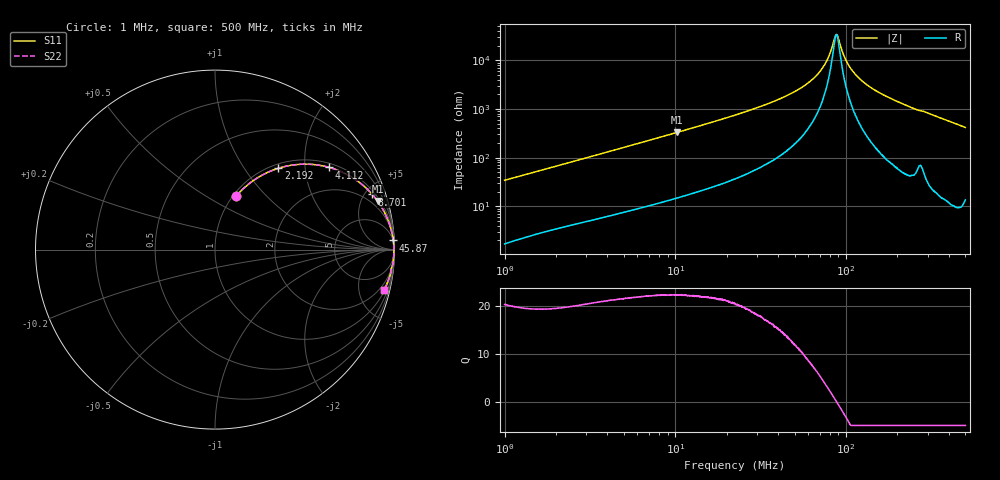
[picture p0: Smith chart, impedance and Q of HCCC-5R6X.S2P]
!s-Parameter Generated by FASTRON Sdn. Bhd.
!FASTRON P/N : HCCC-5R6X
!Keysight Technologies,E4991B,MY54100416,A.01.15
!Date: Thu Apr 02 15:32:48 2026
!Version  : Rev00 Thu Apr 02 15:32:48 2026
!Data & Calibration Information:
!PortZ  Port1:50+j0  Port2:50+j0
!When reading, reference impedance value at option line is always used.
! Remarks : This data is being provided solely for informational purposes.
!Freq	S11	S21	S12	S22
# Hz S dB R 50
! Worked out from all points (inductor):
!   1601 points, 1 MHz to 500 MHz, reference 50 ohm
!   read as one part in series: L = 5.38 uH near 1.032 MHz
!   highest Q = 22.3 at 10.24 MHz (marker M1), where L = 5.12 uH
!   self-resonance near 87.75 MHz
!   S11 on the Smith chart (normalised r, x): 1 MHz: 1.03, +0.68; 2.192 MHz: 1.07, +1.45; 4.112 MHz: 1.13, +2.68; 8.701 MHz: 1.25, +5.60; 45.87 MHz: 4, +39; 500 MHz: 1.27, -8.34
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1000000  -9.92 68.6  -0.61 -18.6  -0.61 -18.6  -9.92 68.6
2191518  -4.81 52.1  -2.05 -35.0  -2.05 -35.0  -4.81 52.1
2820919  -3.55 45.6  -2.91 -41.6  -2.91 -41.6  -3.55 45.6
4111646  -2.11 35.8  -4.66 -51.5  -4.66 -51.5  -2.11 35.8
7957584  -0.74 21.0  -8.92 -66.5  -8.92 -66.5  -0.74 21.0
8701196  -0.64 19.3  -9.59 -68.1  -9.59 -68.1  -0.64 19.3
1.024299e7  -0.49 16.6  -10.85 -70.8  -10.85 -70.8  -0.49 16.6
2.236068e7  -0.13 7.6  -17.60 -79.6  -17.60 -79.6  -0.13 7.6
4.587261e7  -0.05 2.9  -25.82 -82.7  -25.82 -82.7  -0.05 2.9
6.307767e7  -0.03 1.4  -31.99 -81.2  -31.99 -81.2  -0.03 1.4
6.978047e7  -0.03 1.0  -35.15 -78.6  -35.15 -78.6  -0.03 1.0
7.541731e7  -0.03 0.7  -38.55 -74.2  -38.55 -74.2  -0.03 0.7
7.994179e7  -0.03 0.4  -42.29 -66.3  -42.29 -66.3  -0.03 0.4
8.573088e7  -0.03 0.1  -49.11 -32.1  -49.11 -32.1  -0.03 0.1
8.809378e7  -0.03 -0.0  -50.64 3.7  -50.64 3.7  -0.03 -0.0
9.01709e7  -0.03 -0.1  -48.92 33.1  -48.92 33.1  -0.03 -0.1
1.001409e8  -0.03 -0.6  -39.87 72.6  -39.87 72.6  -0.03 -0.6
1.125168e8  -0.03 -1.1  -34.49 80.1  -34.49 80.1  -0.03 -1.1
1.361047e8  -0.03 -1.9  -29.37 83.4  -29.37 83.4  -0.03 -1.9
1.77937e8  -0.04 -3.3  -24.71 83.8  -24.71 83.8  -0.04 -3.3
2.553547e8  -0.09 -5.8  -19.93 81.5  -19.93 81.5  -0.09 -5.8
5e8  -0.31 -13.4  -12.71 74.8  -12.71 74.8  -0.31 -13.4
